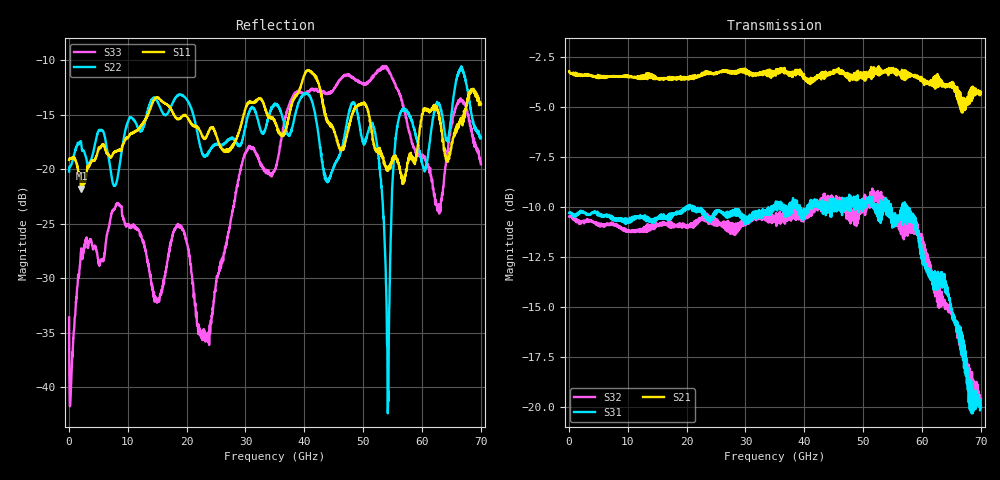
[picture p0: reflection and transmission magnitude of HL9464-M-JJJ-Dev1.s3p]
! 9/8/2020 12:42:44 PM
! H:\PRODUCTION_DATA\TEMP_S3P.S3P
! CHANNEL.1
! TR.MEASUREMENT
! CORRECTED.DATA
# GHZ S RI R 50.0
! FREQ.GHZ  S11RE  S11IM  S12RE  S12IM  S13RE  S13IM
!  S21RE  S21IM  S22RE  S22IM  S23RE  S23IM
!  S31RE  S31IM  S32RE  S32IM  S33RE  S33IM
!; PortSelection: Port_123
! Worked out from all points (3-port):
!   2000 points, 35 MHz to 70 GHz, reference 50 ohm
!   strongest paths, dB at 35 MHz, 17.54 GHz, 35.03 GHz, 52.53 GHz, 70 GHz:
!     S21: -3.2, -3.6, -3.2, -3.4, -4.3
!     S31: -10.3, -10.3, -10.0, -9.9, -20.0
!     S32: -10.5, -10.8, -10.5, -9.3, -19.6
!   lowest |S11| = -21.8 dB at 2.135 GHz (marker M1), VSWR 1.18, Z = 51.1 + j8.18 ohm
!   |S11| at or under -10 dB: start of sweep to end of sweep
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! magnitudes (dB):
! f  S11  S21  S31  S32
! 35 MHz  -19.2  -3.2  -10.3  -10.5
! 2.135 GHz  -21.8  -3.4  -10.2  -10.7
! 18.83 GHz  -15.3  -3.5  -10.2  -10.9
! 23.52 GHz  -16.8  -3.3  -10.6  -10.6
! 29.86 GHz  -14.7  -3.2  -10.7  -10.8
! 35.03 GHz  -15.7  -3.2  -10.0  -10.5
! 51.73 GHz  -17.5  -3.3  -9.8  -9.2
! 54.18 GHz  -19.9  -3.1  -9.9  -9.9
! 56.42 GHz  -20.4  -3.3  -10.5  -11.3
! 70 GHz  -14.1  -4.3  -20.0  -19.6
